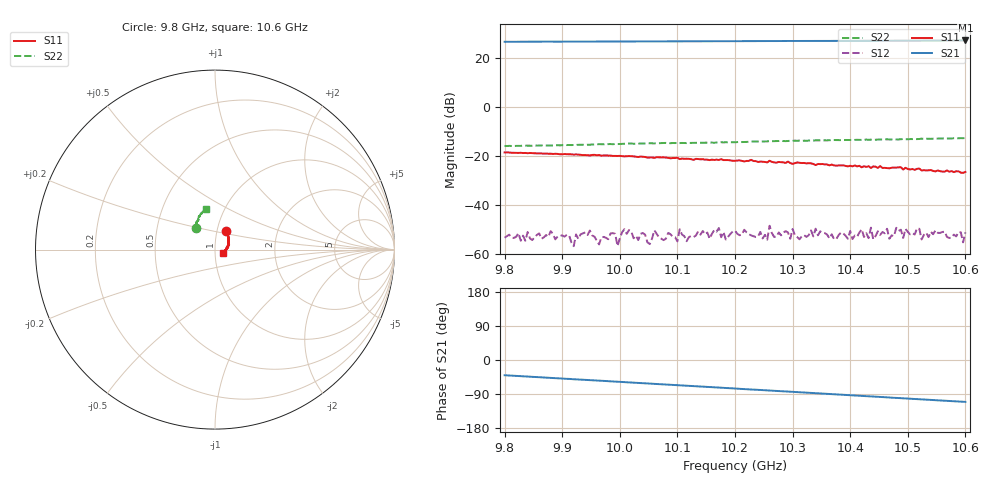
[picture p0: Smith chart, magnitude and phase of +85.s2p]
!Agilent Technologies,E8361C,US49010292,A.09.42.06
!Agilent E8361C: A.09.42.06
!Date: Tuesday, October 15, 2024 23:05:17
!Correction: S11(Full 2 Port(1,2))
!S21(Full 2 Port(1,2))
!S12(Full 2 Port(1,2))
!S22(Full 2 Port(1,2))
!S2P File: Measurements: S11, S21, S12, S22:
# Hz S  dB  R 50
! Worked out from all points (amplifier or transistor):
!   201 points, 9.8 GHz to 10.6 GHz, reference 50 ohm
!   highest |S21| = 27.3 dB at 10.6 GHz (marker M1)
!   |S21| within 3 dB of that: start of sweep to end of sweep
!   unconditionally stable (mu >= 1): start of sweep to end of sweep
!   at 9.932 GHz: K = 8.80, MAG = 27.0 dB, |S12| = -52.0 dB
!   at 10.2 GHz: K = 7.28, MAG = 27.2 dB, |S12| = -50.6 dB
!   at 10.6 GHz: K = 7.47, MAG = 27.5 dB, |S12| = -51.2 dB
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9.8e9  -18.55 59.1  26.72 -40.2  -53.42 52.4  -15.86 130.8
9.88e9  -19.06 52.3  26.77 -47.3  -50.72 59.0  -15.70 128.4
9.92e9  -19.41 48.8  26.78 -50.8  -56.87 55.0  -15.49 127.0
9.936e9  -19.63 47.0  26.80 -52.1  -51.63 38.2  -15.40 126.9
9.964e9  -19.59 45.0  26.80 -54.6  -56.17 51.1  -15.14 125.9
9.992e9  -19.96 42.4  26.83 -57.0  -51.82 46.4  -15.08 125.3
9.996e9  -19.99 39.7  26.84 -57.3  -56.82 50.5  -15.13 124.8
1.0008e10  -20.15 41.3  26.85 -58.5  -49.94 49.7  -14.94 125.0
1.0068e10  -20.53 35.7  26.88 -63.6  -53.29 46.5  -14.76 123.9
1.02e10  -21.97 22.6  26.98 -75.1  -50.56 33.6  -14.39 119.2
1.0336e10  -23.25 7.2  27.08 -87.3  -52.87 39.3  -13.66 114.6
1.0432e10  -24.17 -1.8  27.14 -95.8  -53.59 29.5  -13.38 110.4
1.0436e10  -24.90 -3.2  27.16 -96.1  -49.29 28.2  -13.29 110.7
1.044e10  -24.26 -3.4  27.15 -96.4  -54.06 35.7  -13.35 110.3
1.0464e10  -24.94 -4.1  27.16 -98.6  -49.75 25.5  -13.17 108.9
1.0468e10  -25.04 -9.8  27.18 -98.9  -53.84 34.9  -13.22 109.3
1.048e10  -24.76 -3.9  27.17 -100.0  -49.35 30.7  -13.21 107.8
1.052e10  -25.15 -13.2  27.20 -103.6  -49.77 26.9  -13.04 106.5
1.0524e10  -25.89 -10.9  27.21 -103.9  -54.11 8.3  -12.90 105.7
1.0592e10  -26.78 -22.4  27.23 -110.0  -51.17 27.4  -12.69 103.4
1.0596e10  -26.90 -28.9  27.25 -110.3  -55.31 19.8  -12.71 103.7
1.06e10  -26.50 -24.7  27.26 -110.6  -51.21 22.9  -12.64 102.7
